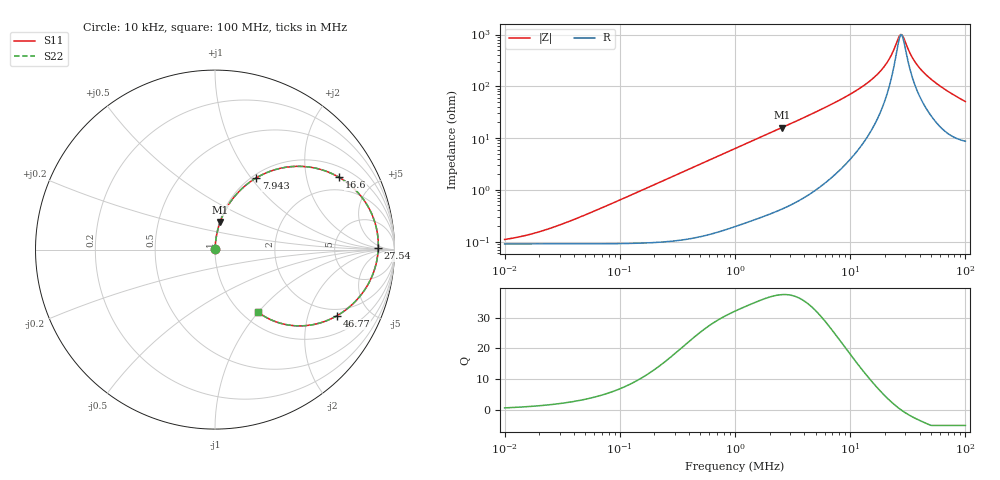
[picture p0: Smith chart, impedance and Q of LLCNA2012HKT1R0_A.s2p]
! LLCNA2012HKT1R0_A  S-PARAMETER MODEL  ( Standard Model )
! Model Generated by TAIYO YUDEN Corporation (http://www.ty-top.com)
! Version 2.0
! TAIYO YUDEN Control No. 171005
! Copyright(c) 2017 TAIYO YUDEN CO.,LTD. All Rights Reserved.
! Product Description (link to TY-COMPAS)
! https://ds.yuden.co.jp/TYCOMPAS/or/detail?pn=LLCNA2012HKT1R0MA&u=M
! Products Name : Inductors
! Characteristics :
!  Inductance : 1.0 [uH] , SRF(min) : - [Hz] , DC Resistance(max) : 111 [mOhm]
!  Rated Current : Saturation  2.26 [A] (dL = 30 [%]), Temp Rise  1.47 [A] (dT = 40 [degC])
!  Case Size : 2.0 x 1.25 / 0.079 x 0.049 [mm/inch] , Thickness : 0.8 / 0.031 [mm/inch]
!  (Conditions: Temperature = 25 [degC] , DC Bias Current = 0 [A])
! External Node Assignments :
!  1  o---GGG---o  2
! GND o---------o GND
! Frequency Range : 10kHz  -  100MHz  [ 402 STEP ]
# MHz S RI R 50
! Freq[MHz].  S11 Real  S11 Imag  S21 Real  S21 Imag  S12 Real  S12 Imag  S22 Real  S22 Imag
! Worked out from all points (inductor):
!   401 points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, 10 kHz to 100 MHz, reference 50 ohm
!   read as one part in series: L = 1 uH near 43.65 kHz
!   highest Q = 37.4 at 2.57 MHz (marker M1), where L = 988 nH
!   self-resonance near 27.78 MHz
!   S11 on the Smith chart (normalised r, x): 10 kHz: 1.00, +0.00; 7.943 MHz: 1.05, +1.06; 16.6 MHz: 1.40, +3.12; 27.54 MHz: 21, +2; 46.77 MHz: 1.69, -3.08; 100 MHz: 1.17, -1.00
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0.01  0.0009 0.000627  0.9991 -0.000627  0.9991 -0.000627  0.0009 0.000627
0.019953  0.000901 0.00125  0.9991 -0.00125  0.9991 -0.00125  0.000901 0.00125
0.046774  0.00091 0.00293  0.9991 -0.00293  0.9991 -0.00293  0.00091 0.00293
0.218776  0.00116 0.0137  0.9988 -0.0137  0.9988 -0.0137  0.00116 0.0137
1  0.00578 0.0618  0.9942 -0.0618  0.9942 -0.0618  0.00578 0.0618
2.570396  0.0288 0.1543  0.9712 -0.1543  0.9712 -0.1543  0.0288 0.1543
4.677351  0.087 0.2672  0.913 -0.2672  0.913 -0.2672  0.087 0.2672
7.943282  0.2291 0.3992  0.7709 -0.3992  0.7709 -0.3992  0.2291 0.3992
12.02264  0.4538 0.4639  0.5462 -0.4639  0.5462 -0.4639  0.4538 0.4639
16.59587  0.6908 0.403  0.3092 -0.403  0.3092 -0.403  0.6908 0.403
19.49845  0.8012 0.3121  0.1988 -0.3121  0.1988 -0.3121  0.8012 0.3121
21.87762  0.862 0.2226  0.138 -0.2226  0.138 -0.2226  0.862 0.2226
26.30268  0.909 0.0524  0.091 -0.0524  0.091 -0.0524  0.909 0.0524
27.54229  0.9097 0.00807  0.0903 -0.00807  0.0903 -0.00807  0.9097 0.00807
28.84032  0.9059 -0.0357  0.0941 0.0357  0.0941 0.0357  0.9059 -0.0357
33.11311  0.8705 -0.1585  0.1295 0.1585  0.1295 0.1585  0.8705 -0.1585
36.30781  0.8304 -0.2295  0.1696 0.2295  0.1696 0.2295  0.8304 -0.2295
40.73803  0.7672 -0.3033  0.2328 0.3033  0.2328 0.3033  0.7672 -0.3033
46.77351  0.6789 -0.3688  0.3211 0.3688  0.3211 0.3688  0.6789 -0.3688
64.56542  0.459 -0.425  0.541 0.425  0.541 0.425  0.459 -0.425
81.28305  0.327 -0.3976  0.673 0.3976  0.673 0.3976  0.327 -0.3976
100  0.2407 -0.3495  0.7593 0.3495  0.7593 0.3495  0.2407 -0.3495
